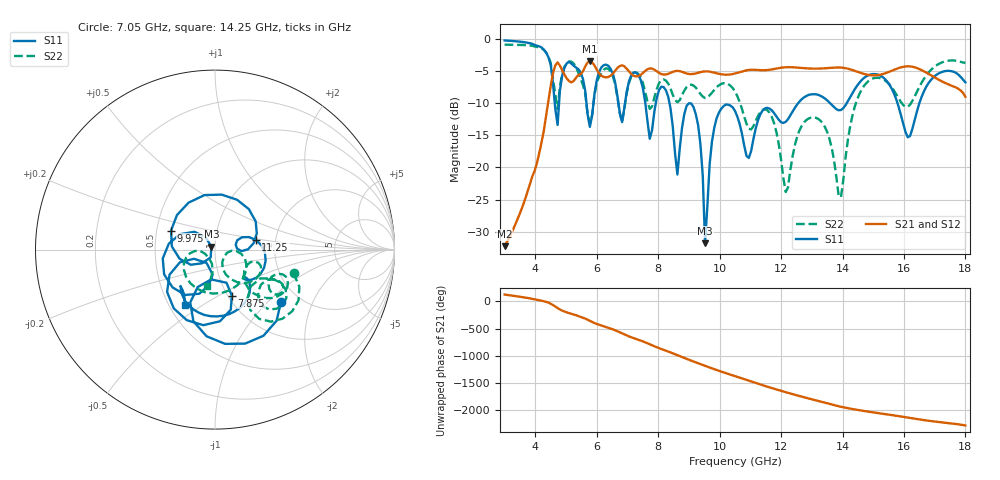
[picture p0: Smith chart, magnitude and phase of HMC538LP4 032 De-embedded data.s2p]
! Chelmsford, MA 01824
! http://www.hittite.com
! Tel: 978-250-3343
! Fax: 978-250-3373
! Device  :  HMC538LP4
! Description:  600 Analog Phase Shifter
! Frequency  :  6.0 GHz - 15.0 GHz
! Package  :  LP4  - 4x4 mm Quad Flatpack No-Lead (QFN) Plastic Package: 24 pin
! Ports  :  2 RF, 1 DC
!  Pin  3  = Rfin  = Port 1
!  Pin  16  = Rfout = Port 2
!  pin  21  = vCTL
! Voltages:  VCTL  = 0 to 5.0 Volts
! Currents :  Vb(V)  Vd(V)  Ib(mA)  Id(mA)
!  0.00  3.20  0.000000	0.468336
! Data:  The device was measured on evaluation board 111296-1.
!  Data was collected using a calibrated network analyzer.
!  The evaluation circuit board was modeled and simulated.This was use
!  to removed the evaluation board circuit from the measured data.
!  The reference plane is the center of the package pin.
! Misc:  Lot #
!Date Measured:  03 - 11 -2009
! Date:  03 - 17 -2009
! Note:
!  Hittite Microwave supplies this data as a sample of measured data at the
!  package pin for this package product.  Your particular data for this product
!  may vary.
!  Data was taken at 25 degrees C.
!  Hittite Microwave reserves the right to change this data at anytime.
# MHz S MA R 50
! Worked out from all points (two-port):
!   201 points, 3 GHz to 18 GHz, reference 50 ohm
!   highest |S21| = -3.47 dB at 5.775 GHz (marker M1); lowest = -32.3 dB at 3 GHz (marker M2)
!   |S21| within 3 dB of the highest: 4.532 GHz to 5.088 GHz (556.7 MHz wide, 11.6 % of centre); 5.258 GHz to 17.19 GHz (11.93 GHz wide, 106 % of centre)
!   lowest |S11| = -31.8 dB at 9.525 GHz (marker M3), VSWR 1.05, Z = 48 + j1.54 ohm
!   |S11| at or under -10 dB: 8.368 GHz to 8.998 GHz (629.6 MHz wide, 7.25 % of centre); 9.023 GHz to 12.55 GHz (3.53 GHz wide, 32.7 % of centre); 15.79 GHz to 16.5 GHz (709.3 MHz wide, 4.39 % of centre)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
!   |S22| runs from -24.6 to -0.9 dB; largest |S21 - S12| = 0.0043
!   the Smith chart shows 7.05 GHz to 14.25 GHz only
!   S11 on the Smith chart (normalised r, x): 7.05 GHz: 1.61, -1.20; 7.875 GHz: 1.04, -0.58; 9.975 GHz: 0.60, +0.14; 11.25 GHz: 1.58, +0.18; 14.25 GHz: 0.60, -0.42
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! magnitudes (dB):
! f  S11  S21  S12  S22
! 3 GHz  -0.2  -32.3  -32.3  -0.9
! 4.65 GHz  -10.9  -4.1  -4.1  -8.6
! 5.55 GHz  -6.2  -5.0  -5.0  -7.2
! 5.775 GHz  -13.7  -3.5  -3.5  -13.2
! 6.15 GHz  -4.4  -5.7  -5.7  -5.3
! 6.825 GHz  -12.9  -4.1  -4.1  -12.9
! 7.05 GHz  -6.6  -5.0  -5.0  -6.8
! 7.875 GHz  -11.3  -4.8  -4.8  -9.1
! 8.025 GHz  -8.0  -5.2  -5.3  -6.9
! 8.625 GHz  -21.1  -4.9  -5.0  -9.8
! 9.225 GHz  -11.7  -5.3  -5.3  -7.6
! 9.525 GHz  -31.8  -5.0  -5.0  -9.2
! 9.975 GHz  -11.5  -5.4  -5.4  -7.2
! 10.5 GHz  -11.2  -5.4  -5.4  -8.1
! 11.25 GHz  -12.6  -4.8  -4.8  -12.0
! 12.15 GHz  -12.9  -4.4  -4.4  -23.8
! 13.05 GHz  -8.6  -4.6  -4.6  -12.2
! 13.95 GHz  -11.0  -4.4  -4.4  -24.6
! 14.25 GHz  -9.0  -4.7  -4.7  -13.6
! 15.53 GHz  -7.1  -5.1  -5.1  -7.1
! 16.12 GHz  -15.3  -4.2  -4.2  -10.5
! 18 GHz  -6.7  -9.0  -9.0  -3.7
